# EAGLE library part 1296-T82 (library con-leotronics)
1.27mm SINGLE ROW FEMALE SOCKET Source: http://www.leotronics.co.uk/Conexcon/Data%20Sheets/sec.%20A/1296ing.pdf
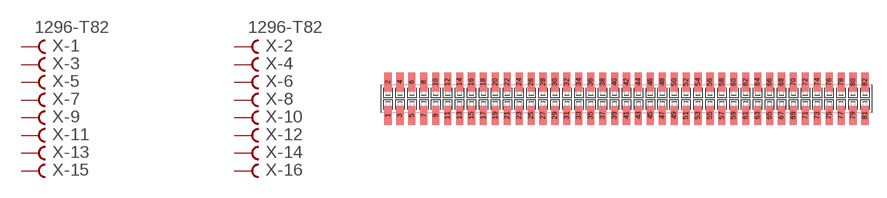
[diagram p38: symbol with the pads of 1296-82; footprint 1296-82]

Designator prefix X; gates -1=FVAL -2=FVAL -3=F -4=F -5=F -6=F -7=F -8=F -9=F -10=F -11=F -12=F -13=F -14=F -15=F -16=F -17=F -18=F -19=F -20=F -21=F -22=F -23=F -24=F -25=F -26=F -27=F -28=F -29=F -30=F -31=F -32=F -33=F -34=F -35=F -36=F -37=F -38=F -39=F -40=F -41=F -42=F -43=F -44=F -45=F -46=F -47=F -48=F -49=F -50=F -51=F -52=F -53=F -54=F -55=F -56=F -57=F -58=F -59=F -60=F -61=F -62=F -63=F -64=F -65=F -66=F -67=F -68=F -69=F -70=F -71=F -72=F -73=F -74=F -75=F -76=F -77=F -78=F -79=F -80=F -81=F -82=F

## 1296-T82 (OC_FARNELL: unknown; OC_NEWARK: unknown)  [1296-82]
1  -1:B  pas
2  -2:B  pas
3  -3:B  pas
4  -4:B  pas
5  -5:B  pas
6  -6:B  pas
7  -7:B  pas
8  -8:B  pas
9  -9:B  pas
10  -10:B  pas
11  -11:B  pas
12  -12:B  pas
13  -13:B  pas
14  -14:B  pas
15  -15:B  pas
16  -16:B  pas
17  -17:B  pas
18  -18:B  pas
19  -19:B  pas
20  -20:B  pas
21  -21:B  pas
22  -22:B  pas
23  -23:B  pas
24  -24:B  pas
25  -25:B  pas
26  -26:B  pas
27  -27:B  pas
28  -28:B  pas
29  -29:B  pas
30  -30:B  pas
31  -31:B  pas
32  -32:B  pas
33  -33:B  pas
34  -34:B  pas
35  -35:B  pas
36  -36:B  pas
37  -37:B  pas
38  -38:B  pas
39  -39:B  pas
40  -40:B  pas
41  -41:B  pas
42  -42:B  pas
43  -43:B  pas
44  -44:B  pas
45  -45:B  pas
46  -46:B  pas
47  -47:B  pas
48  -48:B  pas
49  -49:B  pas
50  -50:B  pas
51  -51:B  pas
52  -52:B  pas
53  -53:B  pas
54  -54:B  pas
55  -55:B  pas
56  -56:B  pas
57  -57:B  pas
58  -58:B  pas
59  -59:B  pas
60  -60:B  pas
61  -61:B  pas
62  -62:B  pas
63  -63:B  pas
64  -64:B  pas
65  -65:B  pas
66  -66:B  pas
67  -67:B  pas
68  -68:B  pas
69  -69:B  pas
70  -70:B  pas
71  -71:B  pas
72  -72:B  pas
73  -73:B  pas
74  -74:B  pas
75  -75:B  pas
76  -76:B  pas
77  -77:B  pas
78  -78:B  pas
79  -79:B  pas
80  -80:B  pas
81  -81:B  pas
82  -82:B  pas

## Footprint 1296-82 (pad centres in mm)
1.27mm SINGLE ROW FEMALE SOCKET Source: http://www.leotronics.co.uk/Conexcon/Data%20Sheets/sec.%20A/1296ing.pdf
smd 0.76 x 2.05: 1 -25.4,-1.78; 2 -25.4,1.78; 3 -24.13,-1.78; 4 -24.13,1.78; 5 -22.86,-1.78; 6 -22.86,1.78; 7 -21.59,-1.78; 8 -21.59,1.78; 9 -20.32,-1.78; 10 -20.32,1.78; 11 -19.05,-1.78; 12 -19.05,1.78; 13 -17.78,-1.78; 14 -17.78,1.78; 15 -16.51,-1.78; 16 -16.51,1.78; 17 -15.24,-1.78; 18 -15.24,1.78; 19 -13.97,-1.78; 20 -13.97,1.78; 21 -12.7,-1.78; 22 -12.7,1.78; 23 -11.43,-1.78; 24 -11.43,1.78; 25 -10.16,-1.78; 26 -10.16,1.78; 27 -8.89,-1.78; 28 -8.89,1.78; 29 -7.62,-1.78; 30 -7.62,1.78; 31 -6.35,-1.78; 32 -6.35,1.78; 33 -5.08,-1.78; 34 -5.08,1.78; 35 -3.81,-1.78; 36 -3.81,1.78; 37 -2.54,-1.78; 38 -2.54,1.78; 39 -1.27,-1.78; 40 -1.27,1.78; 41 0,-1.78; 42 0,1.78; 43 1.27,-1.78; 44 1.27,1.78; 45 2.54,-1.78; 46 2.54,1.78; 47 3.81,-1.78; 48 3.81,1.78; 49 5.08,-1.78; 50 5.08,1.78; 51 6.35,-1.78; 52 6.35,1.78; 53 7.62,-1.78; 54 7.62,1.78; 55 8.89,-1.78; 56 8.89,1.78; 57 10.16,-1.78; 58 10.16,1.78; 59 11.43,-1.78; 60 11.43,1.78; 61 12.7,-1.78; 62 12.7,1.78; 63 13.97,-1.78; 64 13.97,1.78; 65 15.24,-1.78; 66 15.24,1.78; 67 16.51,-1.78; 68 16.51,1.78; 69 17.78,-1.78; 70 17.78,1.78; 71 19.05,-1.78; 72 19.05,1.78; 73 20.32,-1.78; 74 20.32,1.78; 75 21.59,-1.78; 76 21.59,1.78; 77 22.86,-1.78; 78 22.86,1.78; 79 24.13,-1.78; 80 24.13,1.78; 81 25.4,-1.78; 82 25.4,1.78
